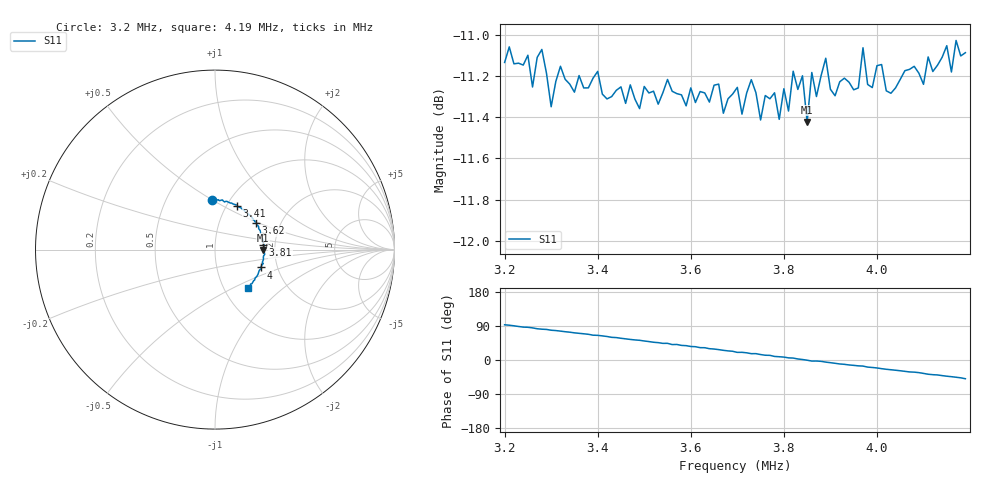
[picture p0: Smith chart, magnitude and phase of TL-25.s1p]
! Touchstone file generated by AntScope (RigExpert AA-54 antenna analyzer)
# MHz Z RI R 50
! Format: Frequency Z-real Z-imaginary (normalized to 50 Ohm)
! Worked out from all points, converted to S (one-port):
!   100 points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, 3.2 MHz to 4.19 MHz, reference 50 ohm
!   lowest |S11| = -11.4 dB at 3.85 MHz (marker M1), VSWR 1.73, Z = 86.7 - j0.5 ohm
!   |S11| at or under -10 dB: start of sweep to end of sweep
!   S11 on the Smith chart (normalised r, x): 3.2 MHz: 0.83, +0.50; 3.41 MHz: 1.11, +0.59; 3.62 MHz: 1.51, +0.48; 3.81 MHz: 1.73, +0.10; 4 MHz: 1.65, -0.35; 4.19 MHz: 1.29, -0.59
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3.2  0.8348 0.5014
3.25  0.8852 0.5338
3.26  0.9026 0.532
3.28  0.9276 0.5562
3.3  0.9592 0.5494
3.33  0.994 0.5702
3.41  1.113 0.5872
3.45  1.187 0.5914
3.55  1.359 0.5616
3.58  1.429 0.5242
3.62  1.506 0.4786
3.7  1.649 0.3358
3.74  1.677 0.2852
3.81  1.732 0.0992
3.82  1.756 0.0936
3.84  1.76 0.0236
3.85  1.734 -0.01
3.86  1.76 -0.0514
3.87  1.746 -0.0486
3.89  1.762 -0.103
3.91  1.728 -0.1538
3.95  1.699 -0.2452
3.97  1.706 -0.286
3.98  1.663 -0.3172
4  1.65 -0.355
4.07  1.527 -0.4776
4.17  1.345 -0.585
4.19  1.29 -0.593
